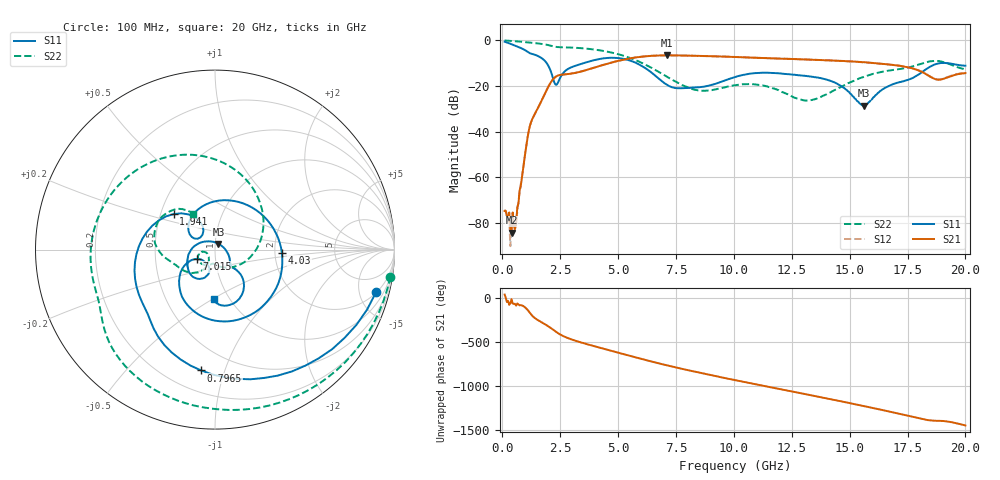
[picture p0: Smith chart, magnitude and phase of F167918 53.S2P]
!  2-Port S-parameters saved by WinCal
! VAR MeasName=S-Parameters (CALIBRATED_DATA) read from VNA (N5242A)
! VAR MeasDate=2016-11-22 10:27:24
! VAR NAME=F167918 53
! VAR FILENAME=F167918 53.S2P
! VAR DATE=2016-11-22 10:27:24
! VAR PHYS_PORTS=1,2
# Hz S DB R 50
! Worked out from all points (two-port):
!   401 points, 100 MHz to 20 GHz, reference 50 ohm
!   highest |S21| = -6.60 dB at 7.115 GHz (marker M1); lowest = -84.2 dB at 398.5 MHz (marker M2)
!   |S21| within 3 dB of the highest: 4.774 GHz to 15.6 GHz (10.83 GHz wide, 106 % of centre)
!   lowest |S11| = -28.6 dB at 15.62 GHz (marker M3), VSWR 1.08, Z = 51.8 + j3.32 ohm
!   |S11| at or under -10 dB: 1.916 GHz to 3.516 GHz (1.599 GHz wide, 58.9 % of centre); 5.793 GHz to 18.92 GHz (13.12 GHz wide, 106 % of centre); 19.21 GHz to end of sweep
!   |S22| runs from -26.4 to -0.1 dB; largest |S21 - S12| = 0.0037
!   S11 on the Smith chart (normalised r, x): 100 MHz: 2.08, -7.12; 796.5 MHz: 0.34, -0.83; 1.941 GHz: 0.58, +0.25; 4.03 GHz: 2.19, -0.09; 7.015 GHz: 0.81, -0.09; 20 GHz: 0.84, -0.51
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1e8  -0.65 -14.8  -74.64 41.0  -74.01 48.8  -0.10 -8.8
3.985e8  -1.73 -52.0  -84.15 -10.5  -78.29 -44.0  -0.30 -33.1
5.975e8  -2.51 -74.7  -80.62 -84.2  -77.32 -74.3  -0.45 -48.6
7.965e8  -3.38 -96.6  -63.87 -78.5  -62.92 -77.7  -0.63 -63.5
1.1945e9  -5.69 -136.2  -37.41 -168.3  -37.36 -168.0  -1.05 -91.1
1.94075e9  -10.35 139.3  -21.25 48.8  -21.22 48.8  -2.02 -136.4
2.33875e9  -19.50 140.4  -15.77 -25.0  -15.74 -24.9  -2.93 -154.3
3.43325e9  -10.26 53.5  -13.59 -145.0  -13.59 -145.0  -3.49 160.3
4.03025e9  -8.56 -2.8  -11.79 171.1  -11.78 171.2  -4.14 133.8
5.42325e9  -8.60 -105.0  -8.12 71.9  -8.07 71.8  -7.41 65.9
6.7665e9  -16.86 -155.8  -6.66 -20.0  -6.67 -20.1  -13.91 -11.7
7.01525e9  -18.86 -152.8  -6.62 -36.0  -6.62 -36.1  -15.36 -26.6
7.11475e9  -19.50 -150.2  -6.60 -42.3  -6.61 -42.4  -15.98 -32.6
8.259e9  -20.68 -120.6  -6.78 -111.0  -6.77 -110.9  -21.52 -87.0
1.005e10  -16.08 -108.0  -7.31 150.2  -7.31 150.2  -19.68 -124.6
1.149275e10  -14.22 -133.2  -7.87 74.6  -7.84 74.4  -20.44 -162.8
1.338325e10  -16.00 -162.7  -8.51 -24.0  -8.49 -24.1  -26.13 -138.5
1.45275e10  -19.43 165.7  -9.01 -84.5  -8.98 -84.7  -20.86 -115.8
1.5622e10  -28.58 59.0  -9.61 -144.4  -9.67 -144.5  -15.97 -126.7
1.67165e10  -19.86 -35.0  -10.59 154.0  -10.64 154.3  -13.25 -150.0
1.8806e10  -10.20 -65.6  -17.27 48.8  -17.13 49.5  -9.06 152.3
2e10  -11.12 -91.6  -14.38 -3.8  -14.26 -3.9  -12.69 121.8
